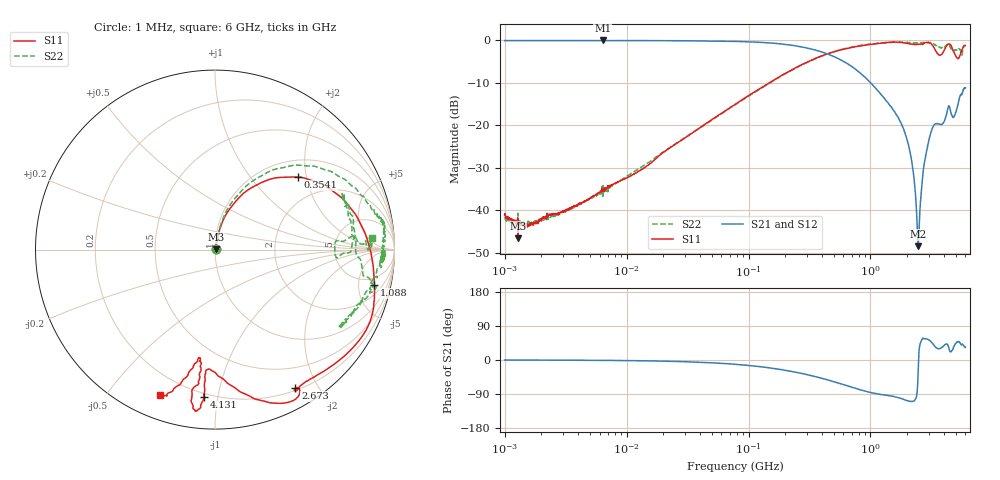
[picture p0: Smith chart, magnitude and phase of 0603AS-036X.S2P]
!s-Parameter Generated by FASTRON Sdn. Bhd.
!FASTRON P/N : 0603AS-036X
!Keysight Technologies: E5071C_MY46733604_B.14.02
!Date: Thu Nov 23 10:58:03 2023
!Version  :Rev01  Thu Nov 23 10:58:03 2023
!Data & Calibration Information:
!Freq  S11:SOLT2(ON)  S21:SOLT2(ON)  S12:SOLT2(ON)  S22:SOLT2(ON)
!PortZ  Port1:50+j0  Port2:50+j0
!When reading reference impedance value at option line is always used.
! Remarks : This data is being provided solely for informational purposes.
# Hz S dB R 50
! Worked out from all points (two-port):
!   1601 points, 1 MHz to 6 GHz, reference 50 ohm
!   highest |S21| = -0.03 dB at 6.378 MHz (marker M1); lowest = -48.4 dB at 2.468 GHz (marker M2)
!   |S21| within 3 dB of the highest: start of sweep to 427.8 MHz
!   lowest |S11| = -46.6 dB at 1.288 MHz (marker M3), VSWR 1.01, Z = 50.4 + j0.229 ohm
!   |S11| at or under -10 dB: start of sweep to 148.5 MHz
!   |S22| runs from -44.0 to -0.4 dB; largest |S21 - S12| = 0.013
!   S11 on the Smith chart (normalised r, x): 1 MHz: 1.02, +0.01; 354.1 MHz: 1.37, +1.78; 1.088 GHz: 3.38, -7.67; 2.673 GHz: 0.23, -1.72; 4.131 GHz: 0.18, -0.91; 6 GHz: 0.11, -0.69
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1000000  -41.03 23.5  -0.05 -0.1  -0.06 -0.1  -41.66 24.1
1287650  -46.62 29.2  -0.07 -0.2  -0.06 -0.1  -40.68 17.1
4277066  -38.37 60.6  -0.07 -0.7  -0.06 -0.7  -38.42 61.0
6378092  -35.33 71.3  -0.03 -1.0  -0.10 -1.1  -36.72 71.9
1.823719e7  -27.32 77.9  -0.08 -2.8  -0.09 -2.8  -27.05 76.6
7.757876e7  -15.08 74.2  -0.25 -11.3  -0.25 -11.2  -15.16 75.6
3.307917e8  -4.63 43.6  -2.07 -41.6  -2.06 -41.6  -4.69 51.2
3.541178e8  -4.25 41.3  -2.30 -44.0  -2.30 -44.0  -4.29 49.1
5.63875e8  -2.27 21.1  -4.53 -62.0  -4.52 -62.0  -2.24 34.6
1.088399e9  -0.83 -12.5  -11.08 -88.2  -11.09 -88.3  -0.80 13.2
1.414819e9  -0.47 -22.1  -15.01 -94.4  -15.02 -94.4  -0.50 9.2
2.024344e9  -0.74 -44.9  -24.08 -107.4  -24.09 -107.3  -0.46 3.2
2.205051e9  -0.93 -52.3  -29.50 -109.3  -29.50 -109.2  -0.52 -1.2
2.379789e9  -0.97 -57.0  -39.77 -97.3  -39.78 -97.0  -0.61 -4.4
2.467691e9  -0.92 -58.4  -48.43 -15.0  -48.53 -15.2  -0.65 -4.4
2.672794e9  -1.00 -59.8  -32.44 57.7  -32.43 57.8  -0.57 -3.7
3.158731e9  -0.87 -70.5  -21.36 47.0  -21.34 47.0  -0.64 -6.2
3.705459e9  -3.52 -93.3  -19.75 30.0  -19.75 29.9  -1.75 -30.0
4.130692e9  -1.67 -94.4  -18.25 41.7  -18.26 41.6  -1.37 -23.0
4.433128e9  -0.87 -97.0  -15.55 26.9  -15.58 26.8  -0.96 -11.7
4.992725e9  -3.67 -97.3  -17.04 43.1  -17.07 43.2  -2.31 21.2
6e9  -1.24 -110.7  -11.19 33.2  -11.18 33.2  -1.12 4.2
